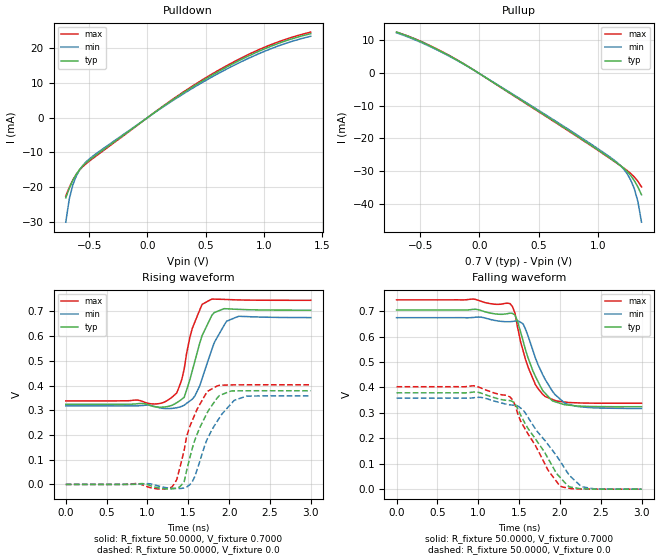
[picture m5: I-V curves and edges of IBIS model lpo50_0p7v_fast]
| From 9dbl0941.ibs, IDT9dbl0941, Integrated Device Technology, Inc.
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|   Model lpo50_0p7v_fast
[Model]  lpo50_0p7v_fast
Model_type Output
Polarity   Non-Inverting
Vmeas =  0.4000V
Cref =   2.0000pF
Rref =   0.0
Vref =   0.4000V
C_comp   1.1000pF   1.0000pF   1.2000pF
[Temperature Range]   27.0000   70.0000   0.0
[Voltage Range]   0.7000V   0.6700V   0.7400V
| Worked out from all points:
|   slope of the pulldown table from 0 to 0.105 V, typ, clamps not added: 41.3 ohm
|   slope of the pullup table from 0 to 0.105 V, typ, clamps not added: 43.4 ohm
|   rising waveform, R_fixture 50.0000, V_fixture 0.7000: 20-80 % time 211ps typ, 243ps min, 174ps max; typ from 0.324 V to 0.705 V
|   rising waveform, R_fixture 50.0000, V_fixture 0.0: 20-80 % time 261ps typ, 298ps min, 232ps max; typ from 0 V to 0.379 V
|   falling waveform, R_fixture 50.0000, V_fixture 0.7000: 20-80 % time 259ps typ, 293ps min, 223ps max; typ from 0.704 V to 0.324 V
|   falling waveform, R_fixture 50.0000, V_fixture 0.0: 20-80 % time 432ps typ, 478ps min, 386ps max; typ from 0.379 V to 0 V
[Pulldown]
|Voltage   I(typ)   I(min)   I(max)
-700mV    -23.07mA   -30.06mA   -22.55mA
-670mV    -20.3mA    -23.39mA   -20.06mA
-640mV    -18.07mA   -19.37mA   -17.97mA
-610mV    -16.28mA   -16.77mA   -16.3mA
-580mV    -14.86mA   -14.94mA   -14.98mA
-550mV    -13.73mA   -13.58mA   -13.94mA
-460mV    -11.23mA   -10.85mA   -11.51mA
200mV     4.757mA    4.547mA    4.904mA
590mV     12.91mA    12.39mA    13.27mA
980mV     19.46mA    18.75mA    19.92mA
1.19V     22.15mA    21.42mA    22.6mA
1.4V      24.16mA    23.42mA    24.62mA
[Pullup]
|Voltage   I(typ)   I(min)   I(max)
-700mV    12.47mA    12.25mA    12.46mA
-430mV    8.493mA    8.28mA     8.576mA
-160mV    3.337mA    3.235mA    3.395mA
590mV     -13.76mA   -13.46mA   -13.9mA
920mV     -21.51mA   -21.16mA   -21.66mA
1.13V     -26.66mA   -26.37mA   -26.76mA
1.22V     -29.12mA   -29.37mA   -29.03mA
1.25V     -30.13mA   -30.86mA   -29.84mA
1.28V     -31.38mA   -32.79mA   -30.73mA
1.31V     -32.94mA   -35.43mA   -31.79mA
1.34V     -34.86mA   -39.33mA   -33.12mA
1.37V     -37.19mA   -45.56mA   -34.8mA
[Ramp]
| variable   typ   min   max
dV/dt_r  0.2273/0.2626n   0.2149/0.2980n   0.2417/0.2521n
dV/dt_f  0.2282/0.2601n   0.2141/0.2926n   0.2441/0.2320n
R_load = 50.0000
[Rising Waveform]
R_fixture= 50.0000
V_fixture= 0.7000
V_fixture_min= 0.6700
V_fixture_max= 0.7400
|time   V(typ)   V(min)   V(max)
0s        324.2mV    317.4mV    337.8mV
1.15ns    312.4mV    309.8mV    327.2mV
1.36ns    330.5mV    310mV      370.6mV
1.42ns    344.4mV    315.8mV    423.7mV
1.52ns    423.9mV    337.5mV    595mV
1.64ns    570.8mV    398.1mV    705mV
1.82ns    695.1mV    574.4mV    749.3mV
1.97ns    710.3mV    660mV      747.9mV
2.12ns    707.8mV    680mV      746.1mV
3ns       704.6mV    674.6mV    744.6mV
[Rising Waveform]
R_fixture= 50.0000
V_fixture= 0.0
V_fixture_min= 0.0
V_fixture_max= 0.0
|time   V(typ)   V(min)   V(max)
0s        578.5nV    0V         711.6nV
1.3ns     -17.82mV   -15.7mV    -10.9mV
1.36ns    -13.96mV   -16.96mV   20.3mV
1.45ns    10.82mV    -14.3mV    138.7mV
1.48ns    55.77mV    -10.98mV   194mV
1.64ns    228.9mV    91.68mV    322.7mV
1.73ns    288.8mV    181.5mV    374.6mV
1.88ns    359mV      268.1mV    400.8mV
2.21ns    378.7mV    356.7mV    402.8mV
3ns       378.8mV    358.1mV    402.8mV
[Falling Waveform]
R_fixture= 50.0000
V_fixture= 0.7000
V_fixture_min= 0.6700
V_fixture_max= 0.7400
|time   V(typ)   V(min)   V(max)
0s        704.5mV    674.4mV    744.6mV
1ns       705.9mV    677.1mV    743.1mV
1.39ns    692.3mV    658.6mV    729.8mV
1.45ns    685.4mV    661mV      692.6mV
1.55ns    582.6mV    650mV      544.1mV
1.7ns     443.9mV    516.2mV    411.5mV
1.82ns    377.3mV    431.4mV    364.4mV
1.94ns    344mV      372.1mV    348.8mV
2.09ns    331mV      334.5mV    341.4mV
3ns       324.2mV    317.5mV    337.8mV
[Falling Waveform]
R_fixture= 50.0000
V_fixture= 0.0
V_fixture_min= 0.0
V_fixture_max= 0.0
|time   V(typ)   V(min)   V(max)
0s        378.8mV    358.1mV    402.8mV
940ps     381.8mV    359.2mV    406.5mV
1.36ns    348.9mV    333.3mV    367.2mV
1.45ns    336.8mV    329.8mV    332.5mV
1.55ns    272.9mV    311.3mV    250.4mV
1.85ns    124mV      177.6mV    77.77mV
2ns       47.23mV    111.5mV    12.69mV
2.12ns    8.387mV    52.94mV    3.191mV
2.27ns    973.9uV    9.45mV     283.3uV
3ns       -59.22uV   -70.17uV   -42.07uV
